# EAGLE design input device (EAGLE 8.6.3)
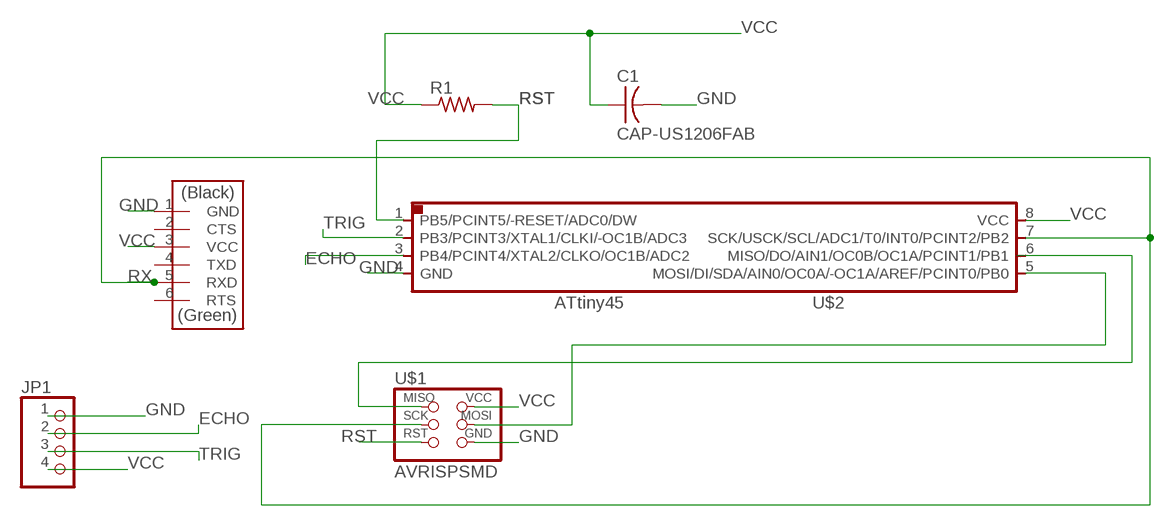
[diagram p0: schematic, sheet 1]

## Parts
C1  CAP-US1206FAB  [C1206FAB]
JP1  PINHD-1X4  [1X04]
R1  RES-US1206FAB  [R1206FAB]
U$1  AVRISPSMD  [2X03SMD]
U$2  ATTINY45SI  [SOIC8]
U$3  FTDI-SMD-HEADER  [1X06SMD]

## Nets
ECHO: JP1.2 U$2.3(PB4/PCINT4/XTAL2/CLKO/OC1B/ADC2)
GND: C1.2 JP1.1 U$1.6(GND) U$2.4(GND) U$3.1(GND)
N$1: U$1.4(MOSI) U$2.5(MOSI/DI/SDA/AIN0/OC0A/-OC1A/AREF/PCINT0/PB0)
N$2: U$1.1(MISO)
RST: R1.2 U$1.5(RST) U$2.1(PB5/PCINT5/-RESET/ADC0/DW)
RX: U$1.3(SCK) U$2.7(SCK/USCK/SCL/ADC1/T0/INT0/PCINT2/PB2) U$3.5(RXD)
TRIG: JP1.3 U$2.2(PB3/PCINT3/XTAL1/CLKI/-OC1B/ADC3)
VCC: C1.1 JP1.4 R1.1 U$1.2(VCC) U$2.8(VCC) U$3.3(VCC)
Unconnected: U$2.6(MISO/DO/AIN1/OC0B/OC1A/PCINT1/PB1) U$3.2(CTS) U$3.4(TXD) U$3.6(RTS)

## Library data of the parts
C1 = fab:CAP-US
JP1 = pinhead:PINHD-1X4: PIN HEADER
R1 = fab:RES-US: Resistor (US Symbol)
U$1 = fab:AVRISP
U$2 = fab:ATTINY45
U$3 = fab:FTDI-SMD-HEADER

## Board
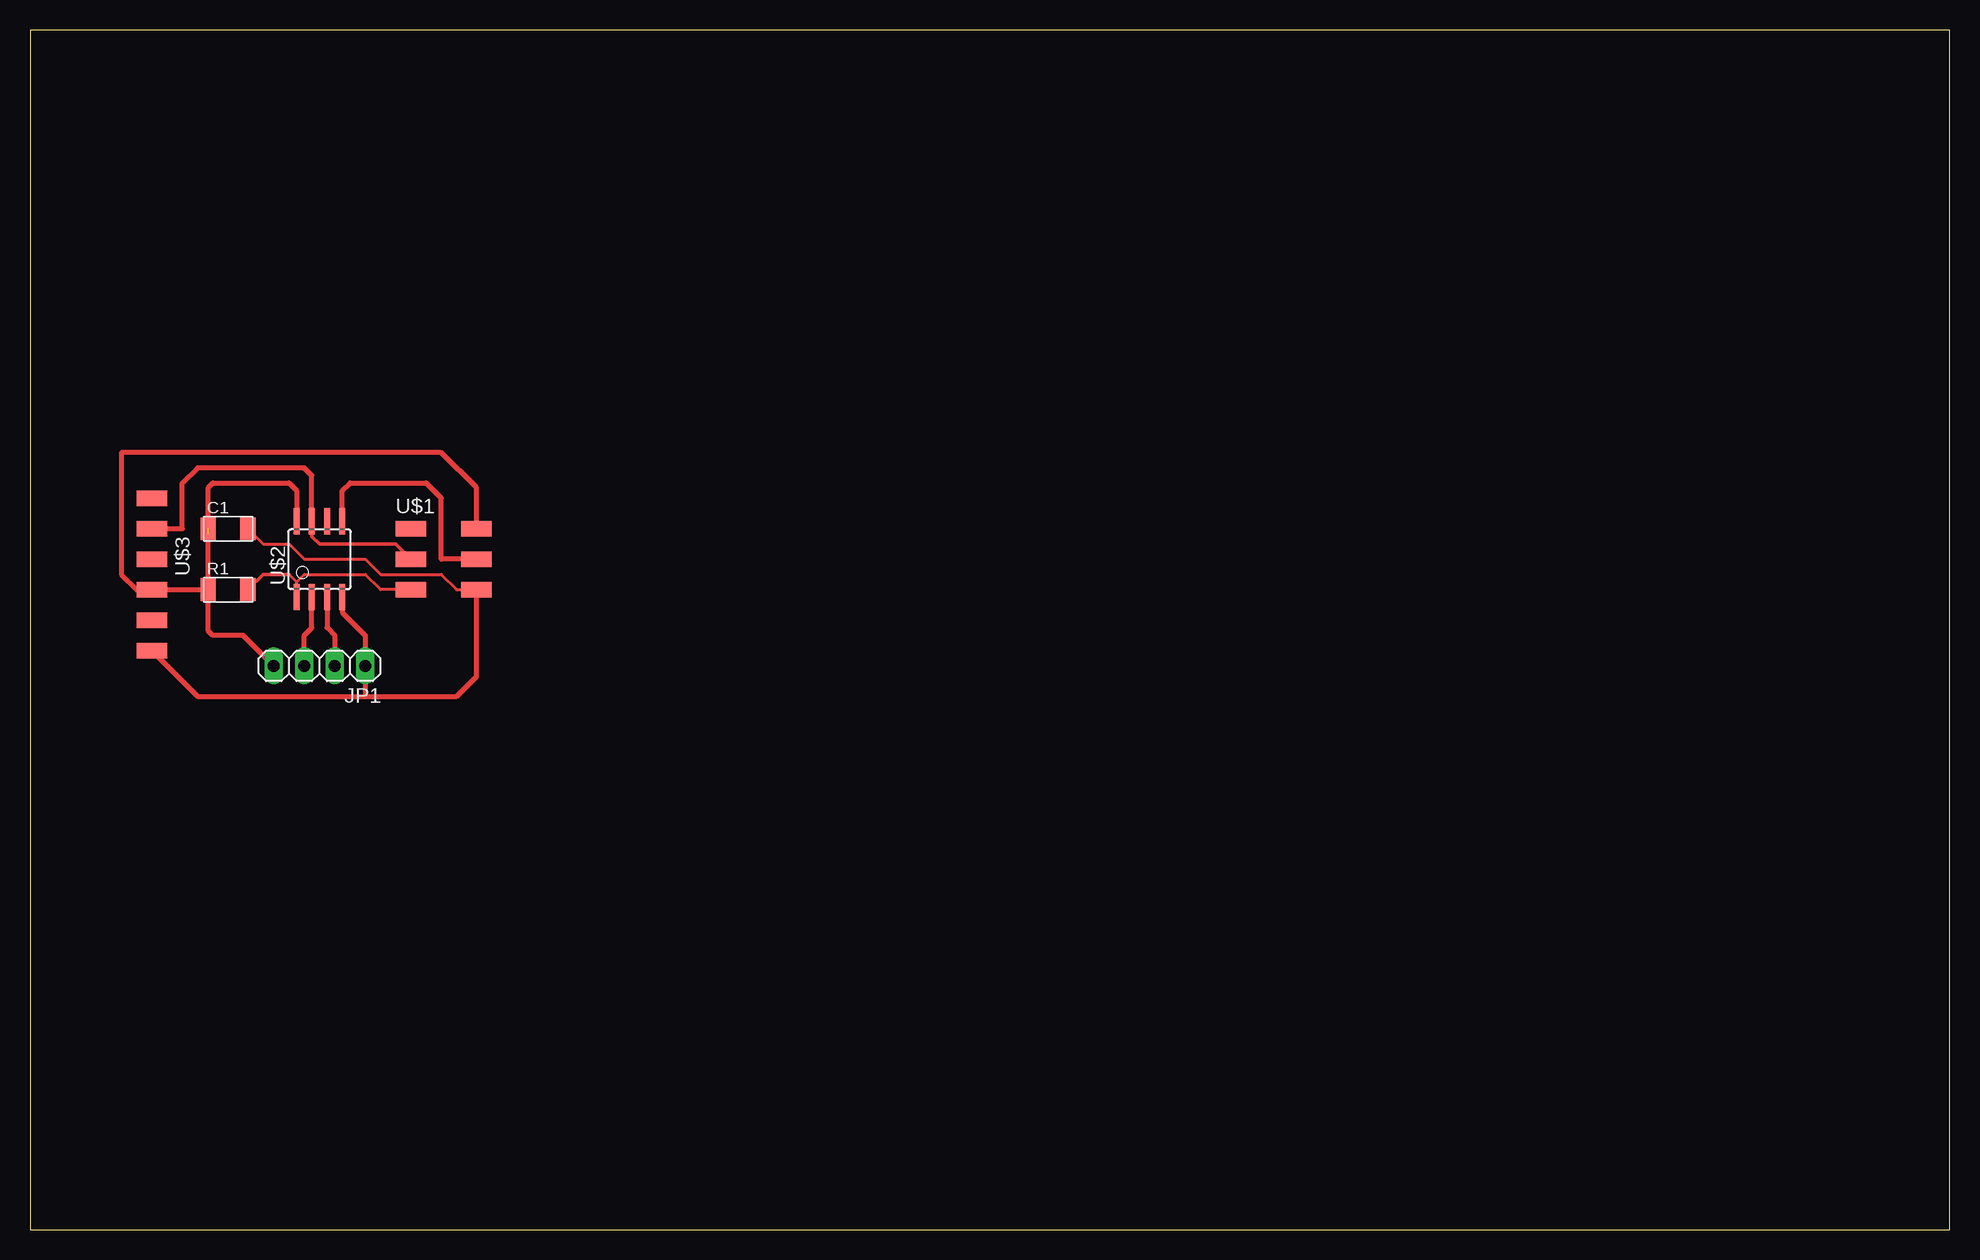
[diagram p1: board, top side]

Size 160 x 100 mm. Coordinates in mm from the lower left corner, seen from the top.
Outline: 0,0 160,0 160,100 0,100 0,0
Copper layers (1*16): Top 0.035mm / dielectric 1.5mm / Bottom 0.035mm
Design rules "default": minimum track width 6mil, minimum drill 0.35mm, track to track 6mil, track to pad 6mil, pad to pad 6mil, via to via 6mil, smd to smd 6mil, copper to edge 40mil, drill to drill 6mil, minimum pad ring 10mil, minimum via ring 8mil, stop-mask expansion 4mil, vias tented up to drill 0mil, thermal gap 10mil

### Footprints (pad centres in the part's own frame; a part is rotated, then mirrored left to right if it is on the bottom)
C1206FAB = smd 1.27 x 1.905: 1 -1.651,0; 2 1.651,0
1X04 = drill 1.016 long: 1 -3.81,0; 2 -1.27,0; 3 1.27,0; 4 3.81,0
R1206FAB = smd 1.27 x 1.905: 1 -1.651,0; 2 1.651,0
2X03SMD = smd 2.54 x 1.27: 1 -2.54,2.54; 2 2.92,2.54; 3 -2.54,0; 4 2.92,0; 5 -2.54,-2.54; 6 2.92,-2.54
SOIC8 = smd 0.5 x 2.2: 1 -1.905,-3.154; 2 -0.645,-3.154; 3 0.625,-3.154; 4 1.895,-3.154; 5 1.905,3.154; 6 0.635,3.154; 7 -0.635,3.154; 8 -1.905,3.154
1X06SMD = smd 2.54 x 1.27: 1 0,6.35; 2 0,3.81; 3 0,1.27; 4 0,-1.27; 5 0,-3.81; 6 0,-6.35

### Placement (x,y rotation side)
C1  16.51,58.42 0 top
JP1  24.13,46.99 180 top
R1  16.51,53.34 0 top
U$1  34.29,55.88 0 top
U$2  24.13,55.88 0 top
U$3  10.16,54.61 180 top

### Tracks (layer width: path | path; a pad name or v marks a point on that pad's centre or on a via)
ECHO
  Top 0.406: U$2.3 24.75,50.17 25.4,49.53 JP1.2
GND
  Top 0.254: C1.2 19.43,57.15 21.59,57.15 22.86,55.88 27.94,55.88 29.21,54.61 34.29,54.61 35.56,53.34 U$1.6
  Top 0.406: U$3.1 13.97,44.45 27.94,44.45 | U$1.6 37.21,46.1 35.56,44.45 27.94,44.45 | 27.94,44.45 JP1.1 27.94,49.53 26.02,51.45 U$2.4
N$1
  Top 0.406: U$1.4 34.29,55.88 34.29,60.96 33.02,62.23 26.67,62.23 26.04,61.59 U$2.5
RST
  Top 0.254: 22.23,53.98 21.59,54.61 | U$2.1 22.23,53.98 | 22.23,53.98 22.86,54.61 27.94,54.61 29.21,53.34 U$1.5
  Top 0.305: 21.59,54.61 19.43,54.61 R1.2
RX
  Top 0.305: U$2.7 23.5,57.78 24.13,57.15 30.48,57.15 U$1.3
  Top 0.406: U$3.5 12.7,58.42 12.7,62.23 13.97,63.5 22.86,63.5 23.5,62.87 U$2.7
TRIG
  Top 0.406: JP1.3 22.86,49.53 23.48,50.16 U$2.2
VCC  (1 unrouted)
  Top 0.406: R1.1 U$3.3 8.89,53.34 7.62,54.61 7.62,64.77 34.29,64.77 37.21,61.85 U$1.2 | R1.1 14.86,58.04 15.24,58.42 | C1.1 14.86,61.85 15.24,62.23 21.59,62.23 22.23,61.59 U$2.8 | JP1.4 17.78,49.53 15.24,49.53 14.86,49.91 R1.1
